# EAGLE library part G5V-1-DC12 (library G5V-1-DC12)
Low Signal Relays - PCB ThruHole Hi-Sens SPDT 12DC 150mW Seal Source: Datasheet
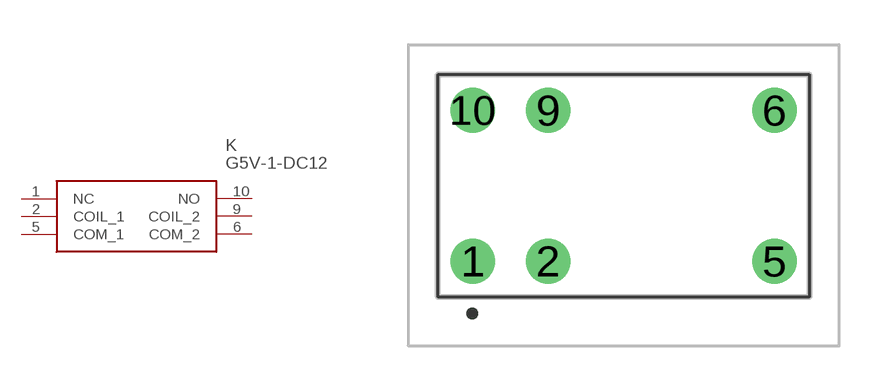
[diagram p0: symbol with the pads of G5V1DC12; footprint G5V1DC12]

Designator prefix K

## G5V-1-DC12 (Allied_Number: 70175802; Description: Low Signal Relays - PCB ThruHole Hi-Sens SPDT 12DC 150mW Seal; Height: 10mm; Manufacturer_Name: Omron Electronics; Manufacturer_Part_Number: G5V-1-DC12)  [G5V1DC12]
1  NC  nc
2  COIL_1  in
5  COM_1
6  COM_2
9  COIL_2  pwr
10  NO  out

## Footprint G5V1DC12 (pad centres in mm)
G5V-1_FFW
drill 1 pad 1.5: 1 -5.08,-2.215; 2 -2.54,-2.215; 5 5.08,-2.215; 6 5.08,2.865; 9 -2.54,2.865; 10 -5.08,2.865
